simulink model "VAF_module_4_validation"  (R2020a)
settings: Solver=VariableStepAuto  StartTime=0.0  StopTime=10.0  RelTol=1e-3
undefined symbols (not defined in the file or in its folder): magnitude

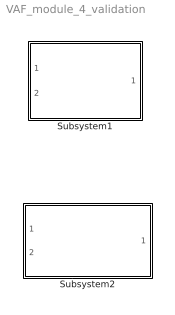
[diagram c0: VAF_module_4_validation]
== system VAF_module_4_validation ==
  Subsystem1 : Subsystem
  Subsystem2 : Subsystem

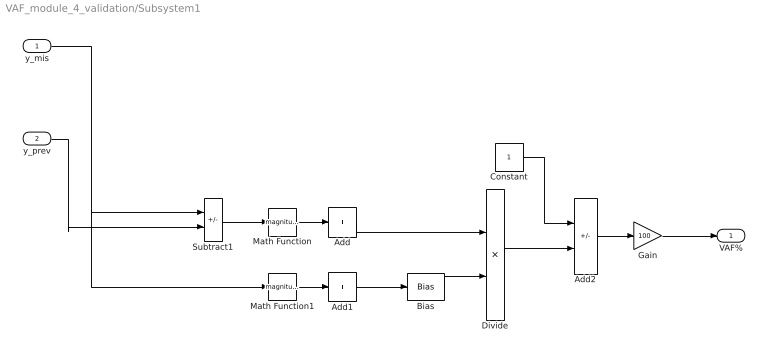
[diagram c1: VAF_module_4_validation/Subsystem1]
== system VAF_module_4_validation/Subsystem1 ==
  y_mis : Inport
  y_prev : Inport  Port=2
  Add : Sum  Inputs=+
  Add1 : Sum  Inputs=+
  Add2 : Sum  Inputs=+-
  Bias : Bias  Bias=1e-7
  Constant : Constant
  Divide : Product  Inputs=*/
  Gain : Gain  Gain=100
  Math Function : Math  Operator=magnitude^2
  Math Function1 : Math  Operator=magnitude^2
  Subtract1 : Sum  Inputs=+-
  VAF% : Outport
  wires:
  Add2/1 -> Gain/1
  Math Function/1 -> Add/1
  Bias/1 -> Divide/2
  y_mis/1 -> Math Function1/1, Subtract1/1
  Add1/1 -> Bias/1
  Math Function1/1 -> Add1/1
  Subtract1/1 -> Math Function/1
  Constant/1 -> Add2/1
  Divide/1 -> Add2/2
  Add/1 -> Divide/1
  y_prev/1 -> Subtract1/2
  Gain/1 -> VAF%/1

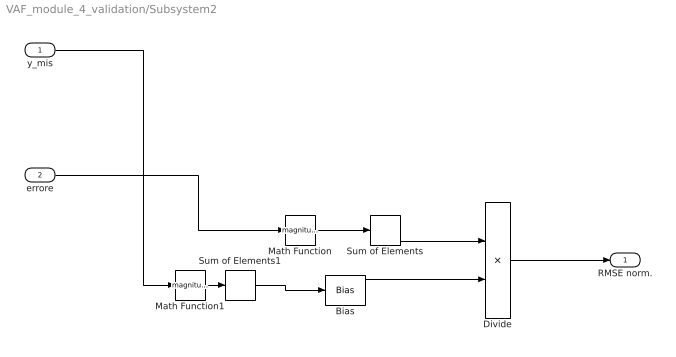
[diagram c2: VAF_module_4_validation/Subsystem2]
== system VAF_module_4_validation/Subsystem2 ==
  y_mis : Inport
  errore : Inport  Port=2
  Bias : Bias  Bias=1e-7
  Divide : Product  Inputs=*/
  Math Function : Math  Operator=magnitude^2
  Math Function1 : Math  Operator=magnitude^2
  Sum of Elements : Sum  Inputs=+
  Sum of Elements1 : Sum  Inputs=+
  RMSE norm. : Outport
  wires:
  Bias/1 -> Divide/2
  Math Function1/1 -> Sum of Elements1/1
  y_mis/1 -> Math Function1/1
  Math Function/1 -> Sum of Elements/1
  errore/1 -> Math Function/1
  Divide/1 -> RMSE norm./1
  Sum of Elements/1 -> Divide/1
  Sum of Elements1/1 -> Bias/1
